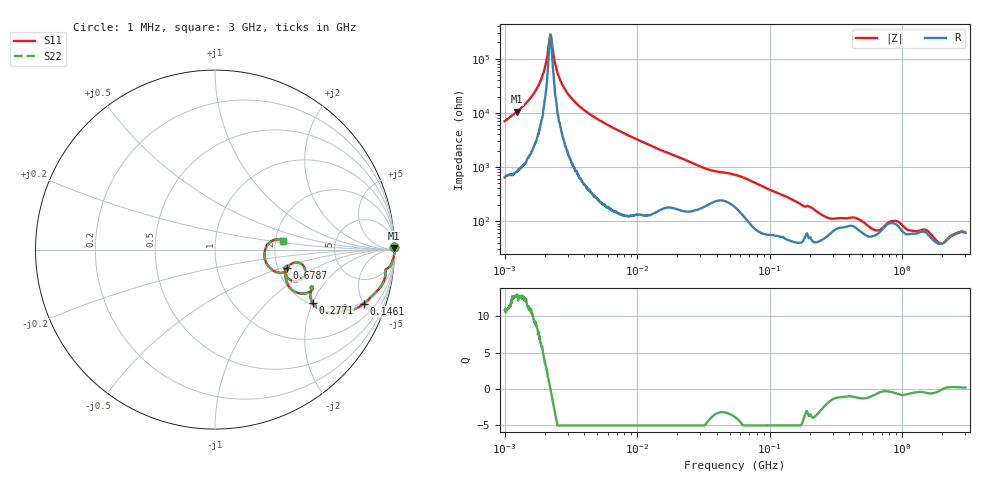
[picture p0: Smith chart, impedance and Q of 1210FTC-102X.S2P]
!s-Parameter Generated by FASTRON Sdn. Bhd.
!FASTRON P/N : 1210FTC-102X
!Keysight Technologies: E4991B_MY54100416_A.01.15
!Date created: Mon Dec 11 09:47:04 2023
!Version  : Rev00 Mon Dec 11 09:47:04 2023
!Data & Calibration Information:
!Freq	S11	S21	S12	S22
!PortZ  Port1:50+j0  Port2:50+j0
!When reading reference impedance value at option line is always used.
! Remarks : This data is being provided solely for informational purposes.
# Hz S dB R 50
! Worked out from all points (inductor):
!   1601 points, 1 MHz to 3 GHz, reference 50 ohm
!   read as one part in series: L = 901 uH near 1.041 MHz
!   highest Q = 12.7 at 1.24 MHz (marker M1), where L = 1.35 mH
!   self-resonance near 2.216 MHz
!   S11 on the Smith chart (normalised r, x): 1 MHz: open; 146.1 MHz: 1.85, -5.01; 277.1 MHz: 2.09, -2.00; 678.7 MHz: 2.25, -0.56; 3 GHz: 2.20, +0.25
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1000000  -0.01 0.8  -36.90 -83.9  -36.90 -83.9  -0.01 0.8
1240074  -0.01 0.5  -40.45 -85.0  -40.45 -85.0  -0.01 0.5
1813890  -0.00 0.2  -50.42 -82.3  -50.42 -82.3  -0.00 0.2
1994811  -0.00 0.1  -55.89 -76.5  -55.89 -76.5  -0.00 0.1
2215843  -0.00 0.0  -68.97 -2.8  -68.97 -2.8  -0.00 0.0
2283380  -0.00 -0.0  -65.31 50.1  -65.31 50.1  -0.00 -0.0
2473713  -0.00 -0.1  -55.78 76.9  -55.78 76.9  -0.00 -0.1
2679912  -0.00 -0.2  -51.13 82.6  -51.13 82.6  -0.00 -0.2
3804036  -0.00 -0.5  -41.79 86.9  -41.79 86.9  -0.00 -0.5
1.447069e7  -0.04 -2.7  -26.63 83.2  -26.63 83.2  -0.04 -2.7
3.320783e7  -0.24 -5.9  -19.56 72.2  -19.56 72.2  -0.24 -5.9
5.477226e7  -0.37 -7.4  -17.47 68.0  -17.47 68.0  -0.37 -7.4
1.460522e8  -1.09 -20.0  -9.18 60.4  -9.18 60.4  -1.09 -20.0
2.083556e8  -2.07 -25.9  -6.93 49.7  -6.93 49.7  -2.07 -25.9
2.771263e8  -4.17 -28.5  -5.29 32.9  -5.29 32.9  -4.17 -28.5
5.337858e8  -5.72 -27.7  -4.55 23.9  -4.55 23.9  -5.72 -27.7
6.787043e8  -7.62 -14.4  -4.35 9.8  -4.35 9.8  -7.62 -14.4
7.925923e8  -6.15 -9.7  -5.66 9.2  -5.66 9.2  -6.15 -9.7
1.01283e9  -6.44 -21.7  -4.66 17.5  -4.66 17.5  -6.44 -21.7
1.542004e9  -7.69 -17.2  -4.18 11.4  -4.18 11.4  -7.69 -17.2
1.970482e9  -11.15 -4.9  -2.80 1.9  -2.80 1.9  -11.15 -4.9
3e9  -8.34 7.4  -4.12 -4.5  -4.12 -4.5  -8.34 7.4
